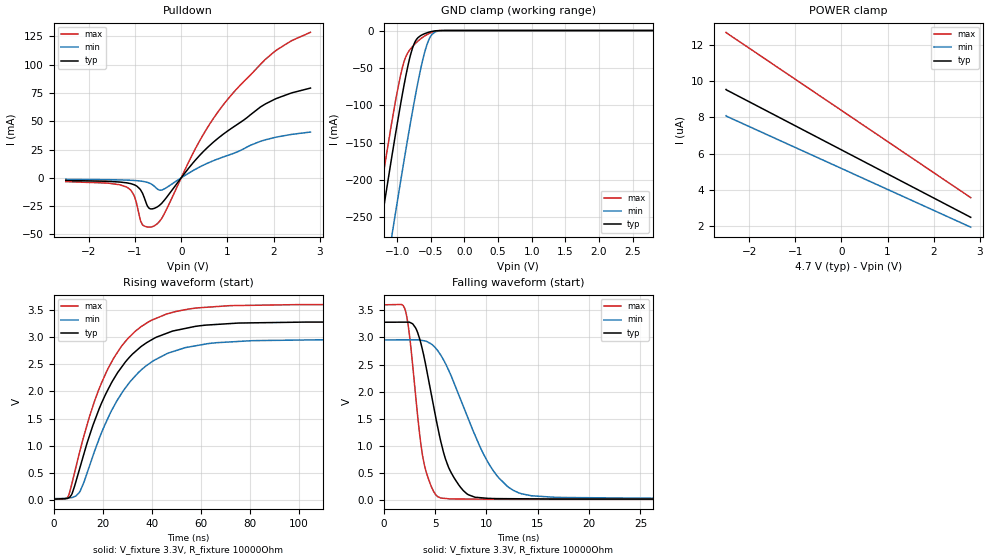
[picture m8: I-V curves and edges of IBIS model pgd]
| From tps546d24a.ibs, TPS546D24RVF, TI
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|   pgd Model
[Model]   pgd
Model_type   I/O_open_drain
Polarity   Inverting
Enable   Active-High
Vinl = 0.8
Vinh = 1.35
Vmeas = 1.65
Vref = 3.3
Cref = 2pF
Rref = 10000
|   typ   min   max
C_comp   2.453pF   2.353pF   2.464pF
|C_comp_pull_down   2.521pF   2.364pF   2.556pF
|  Where Nom  PVT is Nominal Process, 3.3V,   25C
|   Fast PVT is Strong Process,  3.63V, -40C
|   Slow PVT is Weak Process,   2.97V, 150C
[Voltage Range]   3.3   2.97   3.63
|Junction Temperature
[Temperature Range]   25   150   -40
[Pullup Reference]   3.3   2.97   3.63
[Pulldown Reference]   0   0   0
[Power Clamp Reference]   4.7   4.5   4.9
[GND Clamp Reference]   0   0   0
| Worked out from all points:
|   slope of the pulldown table from 0 to 0.495 V, typ, clamps not added: 20.8 ohm
|   GND clamp passes 1 mA (typ) near -0.47 V on its own axis
|   falling waveform, V_fixture 3.3V, R_fixture 10000Ohm: 20-80 % time 2.24ns typ, 4.04ns min, 1.27ns max; typ from 3.28 V to 0.021 V
|   rising waveform, V_fixture 3.3V, R_fixture 10000Ohm: 20-80 % time 19.6ns typ, 20.5ns min, 18.8ns max; typ from 0.021 V to 3.28 V
[Pulldown]
|   Voltage   I(typ)   I(min)   I(max)
-2.5V     -2.272mA   -1.279mA   -3.321mA
-1.175V   -4.431mA   -2.004mA   -8.224mA
-1.016V   -6.131mA   -2.324mA   -16.07mA
-888.8mV  -10.08mA   -2.779mA   -36.71mA
-841.1mV  -13.33mA   -3.038mA   -41.31mA
-698mV    -26.71mA   -4.488mA   -43.56mA
-576.1mV  -26.85mA   -7.631mA   -42.26mA
-406.5mV  -21.76mA   -10.56mA   -34.77mA
383.2mV   19.11mA    9.233mA    31.48mA
976.8mV   40.55mA    19.38mA    67.88mA
2.016V    69.26mA    35.58mA    111.4mA
2.8V      79.32mA    40.49mA    128.6mA
[GND Clamp]
|   Voltage   I(typ)   I(min)   I(max)
-2.5V     -1.021A    -1.121A    -977.8mA
-1.376V   -340.3mA   -447mA     -292.1mA
-1.27V    -278.2mA   -385.1mA   -230.1mA
-1.085V   -172.2mA   -278.5mA   -125.8mA
-1.027V   -140.1mA   -245.5mA   -95.58mA
-904.7mV  -76.85mA   -178.1mA   -43.99mA
-804mV    -33.7mA    -124.7mA   -24.94mA
-735.1mV  -15.34mA   -90.23mA   -17.96mA
-645mV    -6.56mA    -49.54mA   -10.73mA
-517.8mV  -1.986mA   -10.3mA    -3.695mA
-369.4mV  -73.77uA   -390.4uA   -134.2uA
2.8V      0A         0A         0A
[POWER Clamp]
|   Voltage   I(typ)   I(min)   I(max)
-2.5V     9.543uA    8.095uA    12.69uA
-2.495V   9.524uA    8.077uA    12.67uA
-2.299V   9.264uA    7.849uA    12.33uA
2.8V      2.503uA    1.961uA    3.587uA
[Ramp]
R_load = 10000
|   typ   min   max
dV/dt_r   1.95435/1.96749e-08   1.75348/2.05315e-08   2.14872/1.87978e-08
dV/dt_f   1.95436/2.23507e-09   1.75348/4.03531e-09   2.14872/1.26669e-09
[Falling Waveform]
V_fixture = 3.3V
V_fixture_min = 2.97V
V_fixture_max = 3.63V
R_fixture = 10000Ohm
C_fixture = 0F
|   Time   V(typ)   V(min)   V(max)
0s        3.278V     2.953V     3.599V
2.052ns   3.28V      2.954V     3.532V
2.495ns   3.28V      2.955V     3.069V
3.218ns   3.131V     2.955V     1.726V
4.319ns   2.269V     2.911V     415.4mV
6.435ns   560mV      2.349V     26.33mV
8.246ns   102.2mV    1.497V     22.96mV
11.22ns   30.97mV    409.9mV    19.35mV
17.45ns   23.95mV    51.74mV    18.87mV
500ns     21.02mV    30.43mV    17.94mV
[Rising Waveform]
V_fixture = 3.3V
V_fixture_min = 2.97V
V_fixture_max = 3.63V
R_fixture = 10000Ohm
C_fixture = 0F
|   Time   V(typ)   V(min)   V(max)
0s        21.02mV    30.43mV    17.94mV
6.1ns     44.07mV    42.72mV    84.91mV
7.616ns   129.9mV    51.64mV    332.2mV
10.5ns    559.8mV    143.9mV    861.3mV
17.96ns   1.607V     1.056V     1.978V
27.21ns   2.416V     1.928V     2.801V
37.53ns   2.885V     2.466V     3.246V
54.81ns   3.17V      2.816V     3.514V
109.3ns   3.276V     2.951V     3.597V
500ns     3.278V     2.953V     3.599V
